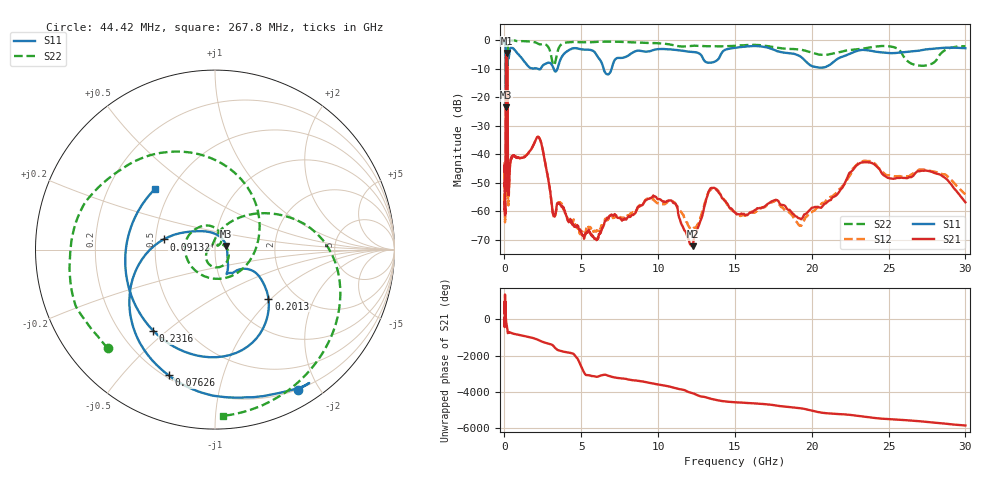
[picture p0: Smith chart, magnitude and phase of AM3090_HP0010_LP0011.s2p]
! Date/Time: Thu, Feb 28, 2019 1:55 PM
! Network Analyzer: Agilent Technologies E8364B Rev: A.07.50.67
! Sweep from 0.010 to 30.000 GHz, 1601 Points, Sweep Type: LOG
! Power Supply: 5.023 V, 0.002 A
# Hz S DB R 50
!freq MagS11 AngS11 MagS21 AngS21 MagS12 AngS12 MagS22 AngS22
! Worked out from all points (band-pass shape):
!   1601 points, 10 MHz to 30 GHz, reference 50 ohm
!   highest |S21| = -4.56 dB at 140.4 MHz (marker M1); lowest = -72.3 dB at 12.25 GHz (marker M2)
!   |S21| within 3 dB of the highest: 100.5 MHz to 188 MHz (87.5 MHz wide, 60.6 % of centre)
!   lowest |S11| = -23.6 dB at 99.43 MHz (marker M3), VSWR 1.14, Z = 56.7 + j2.23 ohm
!   |S11| at or under -10 dB: 2.131 GHz to 2.36 GHz (229.6 MHz wide, 10.2 % of centre); 3.197 GHz to 3.454 GHz (257 MHz wide, 7.73 % of centre); 6.451 GHz to 6.981 GHz (530.3 MHz wide, 7.9 % of centre)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
!   |S22| runs from -31.8 to -0.2 dB; largest |S21 - S12| = 0.01
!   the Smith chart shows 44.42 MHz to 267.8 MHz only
!   S11 on the Smith chart (normalised r, x): 44.42 MHz: 0.19, -1.74; 76.26 MHz: 0.21, -0.67; 91.32 MHz: 0.55, +0.07; 201.3 MHz: 1.48, -0.96; 231.6 MHz: 0.34, -0.45; 267.8 MHz: 0.41, +0.36
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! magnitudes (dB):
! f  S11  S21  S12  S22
! 10 MHz  -0.3  -46.0  -43.1  -0.5
! 38.04 MHz  -0.5  -60.0  -63.4  -1.4
! 44.42 MHz  -0.8  -59.3  -54.8  -1.8
! 76.26 MHz  -2.5  -45.1  -45.0  -4.8
! 91.32 MHz  -10.7  -15.2  -15.2  -15.7
! 99.43 MHz  -23.6  -8.0  -8.0  -15.6
! 140.4 MHz  -16.2  -4.6  -4.5  -24.1
! 144.7 MHz  -16.0  -4.6  -4.5  -22.0
! 179.4 MHz  -14.2  -6.1  -6.1  -31.2
! 201.3 MHz  -7.9  -14.5  -14.4  -11.3
! 231.6 MHz  -4.9  -53.4  -52.7  -1.6
! 267.8 MHz  -6.5  -53.3  -54.9  -0.7
! 550.5 MHz  -2.9  -40.5  -40.5  -0.3
! 2.084 GHz  -10.0  -34.4  -34.4  -1.0
! 3.22 GHz  -10.3  -61.2  -62.3  -8.9
! 7.926 GHz  -5.9  -62.9  -61.9  -0.7
! 9.878 GHz  -3.3  -55.1  -56.9  -1.1
! 12.25 GHz  -4.2  -72.3  -66.2  -2.0
! 13.68 GHz  -7.6  -51.9  -52.1  -2.2
! 19.61 GHz  -7.5  -61.0  -62.0  -3.8
! 23.36 GHz  -3.5  -42.9  -42.4  -3.0
! 30 GHz  -2.9  -56.9  -54.1  -2.2
